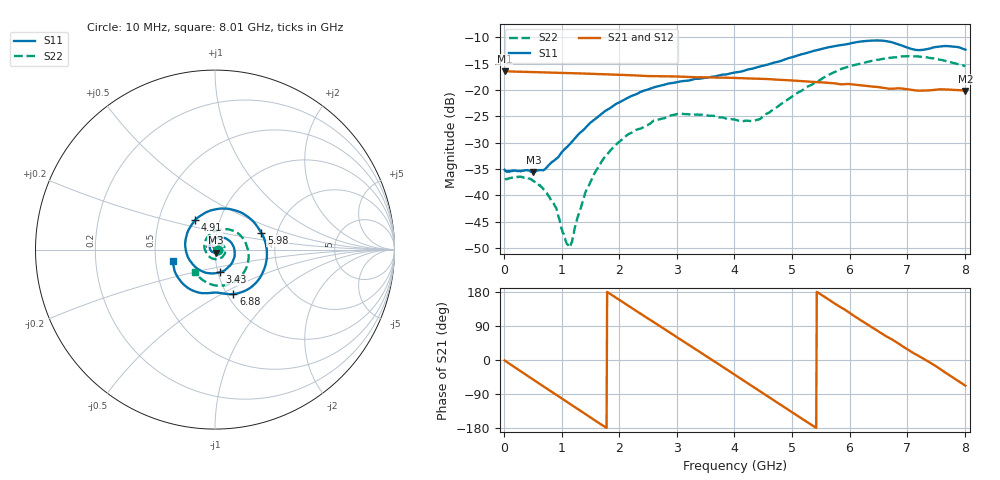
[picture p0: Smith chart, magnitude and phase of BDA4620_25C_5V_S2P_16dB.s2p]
!Agilent Technologies,E5071B,MY42404982,A.09.10
!Date: Wed May 06 09:01:37 2026
!Data & Calibration Information:
!Freq	S11:SOLT2(ON)	S21:SOLT2(ON)	S12:SOLT2(ON)	S22:SOLT2(ON)
# Hz S RI R 50
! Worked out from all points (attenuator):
!   801 points, 10 MHz to 8.01 GHz, reference 50 ohm
!   highest |S21| = -16.43 dB at 10 MHz (marker M1); lowest = -20.2 dB at 8.01 GHz (marker M2)
!   lowest |S11| = -35.6 dB at 510 MHz (marker M3), VSWR 1.03, Z = 50.3 - j1.65 ohm
!   |S11| at or under -10 dB: start of sweep to end of sweep
!   |S22| runs from -49.7 to -13.6 dB; largest |S21 - S12| = 0.00072
!   S11 on the Smith chart (normalised r, x): 10 MHz: 1.04, -0.00; 3.43 GHz: 1.03, -0.26; 4.91 GHz: 0.76, +0.26; 5.98 GHz: 1.66, +0.33; 6.88 GHz: 1.07, -0.57; 8.01 GHz: 0.62, -0.08
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1e7  0.0174 -0.00134  0.1509 -0.00318  0.1511 -0.00324  0.0142 -0.000526
5.1e8  0.00309 -0.0164  0.0911 -0.1168  0.0912 -0.1171  0.0121 -0.00631
8.8e8  -0.0191 -0.01  0.0016 -0.1462  0.00141 -0.1465  0.00311 -0.00731
1.12e9  -0.0289 0.00691  -0.0578 -0.1329  -0.0581 -0.1331  -0.00265 -0.00195
1.18e9  -0.0297 0.0126  -0.0713 -0.1257  -0.0715 -0.126  -0.00358 4.73e-05
1.35e9  -0.0286 0.0287  -0.1043 -0.0987  -0.1044 -0.0989  -0.00544 0.00604
1.58e9  -0.0162 0.0503  -0.1331 -0.0498  -0.1333 -0.0498  -0.00434 0.0159
1.87e9  0.0157 0.0672  -0.1388 0.0203  -0.1391 0.0204  0.00457 0.0271
2.16e9  0.0564 0.0636  -0.1105 0.0837  -0.1105 0.0837  0.0201 0.0322
2.68e9  0.1088 -0.00195  -0.00449 0.1351  -0.00445 0.1354  0.049 0.0186
3.43e9  0.0292 -0.1255  0.1256 0.0412  0.1258 0.0411  0.0428 -0.0395
4.01e9  -0.1106 -0.0962  0.1006 -0.0826  0.1007 -0.0828  -0.0161 -0.0498
4.42e9  -0.1654 0.0132  0.0221 -0.1258  0.0221 -0.126  -0.0513 -0.0116
4.91e9  -0.1102 0.1653  -0.0779 -0.0964  -0.078 -0.0967  -0.0441 0.067
5.35e9  0.0429 0.2291  -0.1186 -0.0159  -0.1187 -0.0159  0.0254 0.1101
5.98e9  0.2588 0.0923  -0.0678 0.0919  -0.0678 0.0919  0.153 0.0663
6.33e9  0.2848 -0.0709  -0.00343 0.1087  -0.00336 0.1088  0.1857 -0.0103
6.68e9  0.1888 -0.218  0.0532 0.0879  0.0534 0.0883  0.1751 -0.0998
6.88e9  0.1021 -0.248  0.0791 0.067  0.0793 0.0672  0.1486 -0.1453
7.19e9  0.00599 -0.2389  0.0967 0.0194  0.097 0.0196  0.0755 -0.1945
7.55e9  -0.1127 -0.2325  0.0943 -0.0372  0.0944 -0.0373  -0.02 -0.1937
8.01e9  -0.2326 -0.0646  0.037 -0.0909  0.0372 -0.0911  -0.1139 -0.1238
